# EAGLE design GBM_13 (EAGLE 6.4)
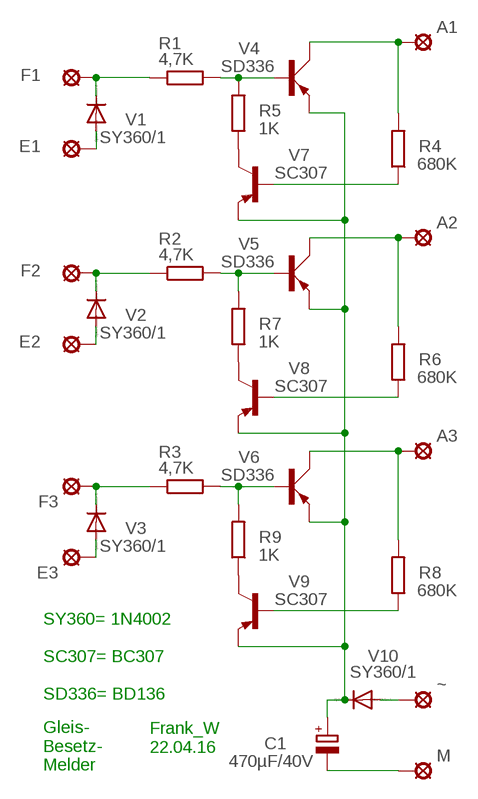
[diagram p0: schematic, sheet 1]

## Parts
A1  LSP10  [LSP10]
A2  LSP10  [LSP10]
A3  LSP10  [LSP10]
C1  470µF/40V  CPOL-EUE22-9AXIAL  [E22-9]
E1  LSP10  [LSP10]
E2  LSP10  [LSP10]
E3  LSP10  [LSP10]
F1  LSP10  [LSP10]
F2  LSP10  [LSP10]
F3  LSP10  [LSP10]
M  LSP10  [LSP10]
R1  4,7K  R-EU_0207/12  [0207/12]
R2  4,7K  R-EU_0207/12  [0207/12]
R3  4,7K  R-EU_0207/12  [0207/12]
R4  680K  R-EU_0207/12  [0207/12]
R5  1K  R-EU_0207/12  [0207/12]
R6  680K  R-EU_0207/12  [0207/12]
R7  1K  R-EU_0207/12  [0207/12]
R8  680K  R-EU_0207/12  [0207/12]
R9  1K  R-EU_0207/12  [0207/12]
V1  SY360/1  1N4004  [DO41-10]
V2  SY360/1  1N4004  [DO41-10]
V3  SY360/1  1N4004  [DO41-10]
V4  SD336  BD140  [TO126AV]
V5  SD336  BD140  [TO126AV]
V6  SD336  BD140  [TO126AV]
V7  SC307  BC307  [TO92]
V8  SC307  BC307  [TO92]
V9  SC307  BC307  [TO92]
V10  SY360/1  1N4004  [DO41-10]
~  LSP10  [LSP10]

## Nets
N$1: E1.MP V1.A
N$2: F1.MP R1.1 V1.C
N$3: R1.2 R5.2 V4.B
N$4: A1.MP R4.2 V4.C
N$5: R4.1 V7.2(B)
N$6: R5.1 V7.3(C)
N$7: F2.MP R2.1 V2.C
N$8: E2.MP V2.A
N$9: R2.2 R7.2 V5.B
N$10: R7.1 V8.3(C)
N$11: A2.MP R6.2 V5.C
N$12: R6.1 V8.2(B)
N$13: R9.1 V9.3(C)
N$14: F3.MP R3.1 V3.C
N$15: R3.2 R9.2 V6.B
N$16: A3.MP R8.2 V6.C
N$17: R8.1 V9.2(B)
N$18: E3.MP V3.A
N$19: V10.A ~.MP
N$20: C1.- M.MP
N$21: C1.+ V4.E V5.E V6.E V7.1(E) V8.1(E) V9.1(E) V10.C

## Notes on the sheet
- SY360= 1N4002
  
  SC307= BC307
  
  SD336= BD136
- Frank_W
  22.04.16
- Gleis-
  Besetz-
  Melder

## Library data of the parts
A1-A3 E1-E3 F1-F3 M ~ = solpad:LSP10: SOLDER PAD
C1 = rcl:CPOL-EU: POLARIZED CAPACITOR, European symbol
R1-R9 = rcl:R-EU_: RESISTOR, European symbol
V1-V3 V10 = diode:1N4004: DIODE
V4-V6 = transistor-power:BD140: PNP TRANSISTOR
V7-V9 = transistor-pnp:BC307: PNP Transistor

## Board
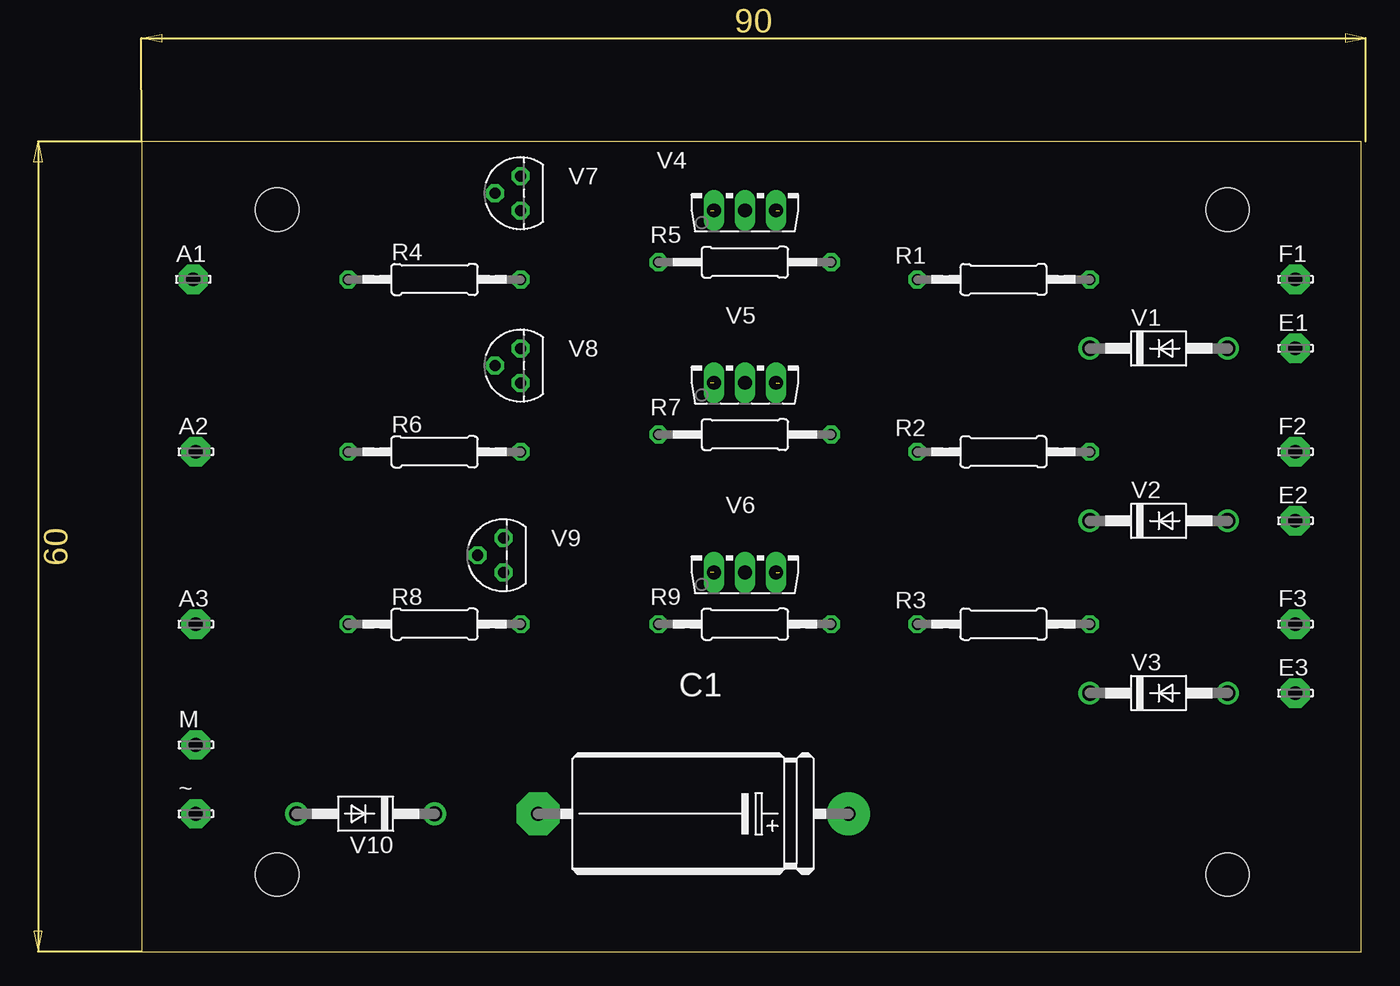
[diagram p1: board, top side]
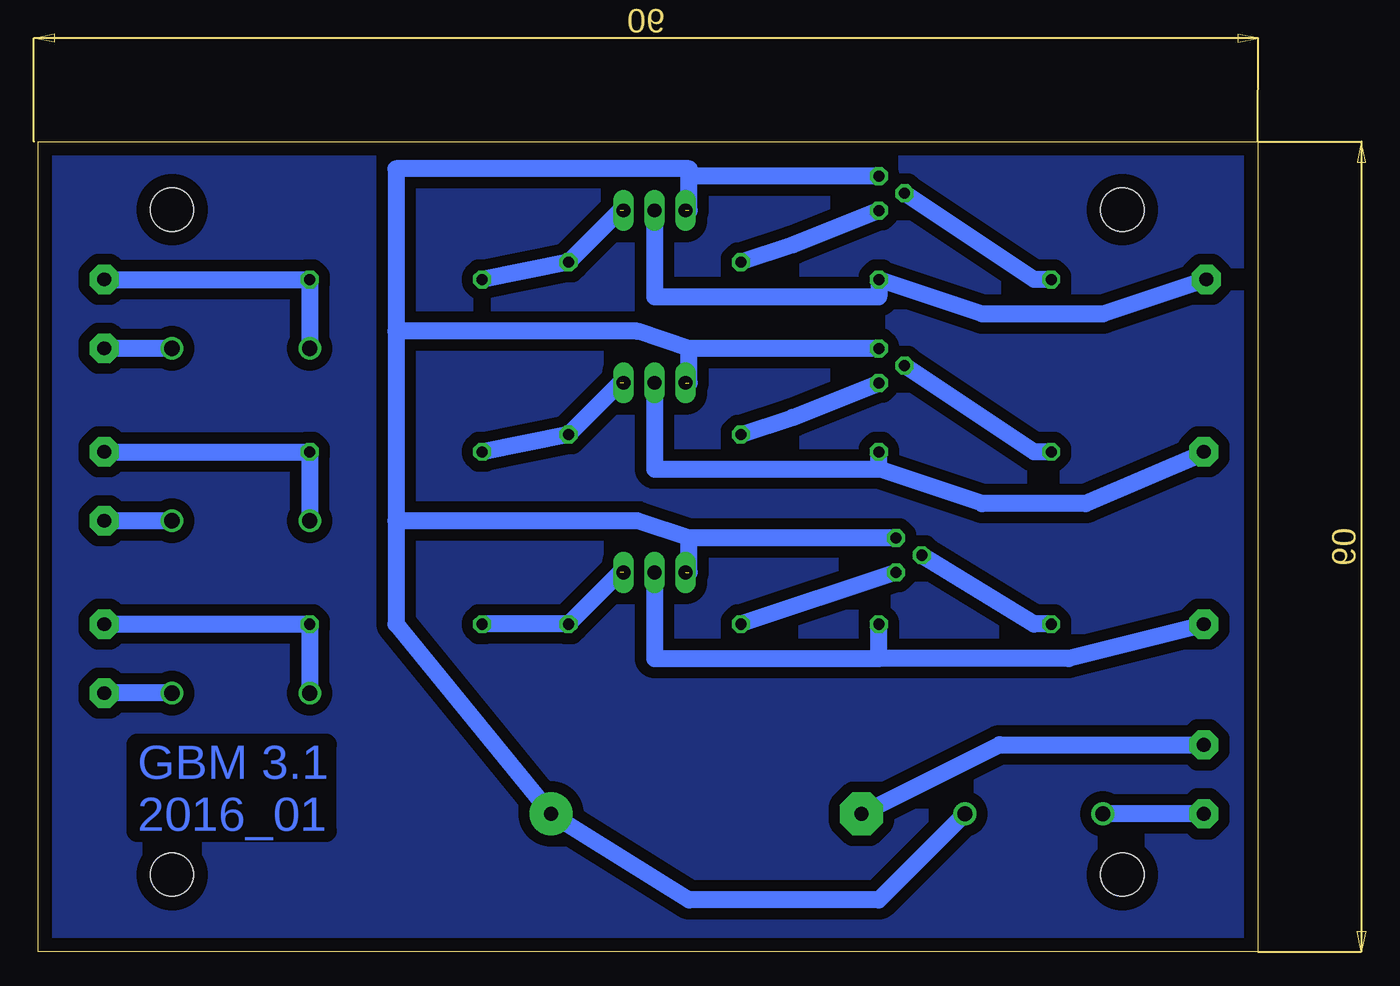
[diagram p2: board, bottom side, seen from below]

Size 98.09 x 67.61 mm. Coordinates in mm from the lower left corner, seen from the top.
Outline: 7.92,0 97.76,0 97.76,59.68 7.92,59.68 7.92,0
Copper layers (1*16): Top 0.035mm / dielectric 1.5mm / Bottom 0.035mm
Design rules "default *": minimum track width 20mil, minimum drill 24mil, track to track 8mil, track to pad 8mil, pad to pad 8mil, via to via 8mil, smd to smd 8mil, copper to edge 40mil, drill to drill 8mil, minimum pad ring 10mil, minimum via ring 8mil, stop-mask expansion 4mil, vias tented up to drill 0mil, thermal gap 20mil
Holes 3.2 mm at 87.92,54.68 87.92,5.68 17.92,5.68 17.92,54.68

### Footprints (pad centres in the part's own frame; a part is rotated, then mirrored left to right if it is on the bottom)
LSP10 = drill 1.016 pad 2.159 octagon: MP 0,0
E22-9 = drill 1.016 pad 3.15: + -11.43,0 | drill 1.016 pad 3.15 octagon: - 11.43,0
0207/12 = drill 0.813 octagon: 1 -6.35,0; 2 6.35,0
DO41-10 = drill 1.118: A 5.08,0; C -5.08,0
TO126AV = drill 1.016 long: B 2.286,-1.27; C 0,-1.27; E -2.286,-1.27
TO92 = drill 0.813 octagon: 1 1.27,0; 2 0,1.905; 3 -1.27,0

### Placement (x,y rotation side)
A1  11.73,49.53 0 top
A2  11.92,36.83 0 top
A3  11.92,24.13 0 top
C1  48.56,10.16 180 top
E1  92.92,44.45 0 top
E2  92.92,31.75 0 top
E3  92.92,19.05 0 top
F1  92.92,49.53 0 top
F2  92.92,36.83 0 top
F3  92.92,24.13 0 top
M  11.92,15.24 0 top
R1  71.42,49.53 180 top
R2  71.42,36.83 180 top
R3  71.42,24.13 180 top
R4  29.51,49.53 0 top
R5  52.37,50.8 0 top
R6  29.51,36.83 0 top
R7  52.37,38.1 0 top
R8  29.51,24.13 0 top
R9  52.37,24.13 0 top
V1  82.85,44.45 0 top
V2  82.85,31.75 0 top
V3  82.85,19.05 0 top
V4  52.37,55.88 0 top
V5  52.37,43.18 0 top
V6  52.37,29.21 0 top
V7  35.86,55.88 90 top
V8  35.86,43.18 90 top
V9  34.59,29.21 90 top
V10  24.43,10.16 180 top
~  11.92,10.16 0 top

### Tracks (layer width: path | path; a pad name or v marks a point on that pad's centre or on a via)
N$1
  Bottom 1.27: V1.A E1.MP
N$2
  Bottom 1.27: F1.MP R1.1 V1.C
N$3  (1 unrouted)
  Bottom 1.27: 54.91,54.61 R5.2 R1.2
N$4
  Bottom 1.27: A1.MP 19.35,46.99 28.24,46.99 R4.2 35.86,48.26 52.37,48.26 V4.C
N$5
  Bottom 1.27: R4.1 24.43,49.53 V7.2
N$6
  Bottom 1.27: V7.3 42.21,52.07 R5.1
N$7
  Bottom 1.27: F2.MP R2.1 V2.C
N$8
  Bottom 1.27: V2.A E2.MP
N$9  (1 unrouted)
  Bottom 1.27: 54.91,41.91 R7.2 R2.2
N$10
  Bottom 1.27: R7.1 42.21,39.37 V8.3
N$11
  Bottom 1.27: 35.86,35.56 52.37,35.56 V5.C | 35.86,35.56 R6.2 | A2.MP 11.73,36.83 20.62,33.02 28.24,33.02 35.86,35.56
N$12
  Bottom 1.27: R6.1 24.43,36.83 V8.2
N$13
  Bottom 1.27: V9.3 R9.1
N$14
  Bottom 1.27: F3.MP R3.1 V3.C
N$15  (1 unrouted)
  Bottom 1.27: 54.91,27.94 R9.2 R3.2
N$16
  Bottom 1.27: 35.86,21.59 52.37,21.59 V6.C | 35.86,21.59 R8.2 | A3.MP 11.73,24.13 21.89,21.59 35.86,21.59
N$17
  Bottom 1.27: R8.1 24.43,24.13 V9.2
N$18
  Bottom 1.27: V3.A E3.MP
N$19
  Bottom 1.27: ~.MP V10.A
N$20
  Bottom 1.27: C1.- 26.97,15.24 M.MP
N$21  (3 unrouted)
  Bottom 1.27: V10.C 35.86,3.81 49.83,3.81 C1.+ 71.42,24.13 71.42,31.75 | 49.83,54.61 49.83,57.15 | 71.42,45.72 71.42,57.68 49.83,57.68 49.83,57.15 | 71.42,45.72 71.42,31.75 | V7.1 49.83,57.15 | 49.83,41.91 49.83,44.45 | 49.83,44.45 53.64,45.72 71.42,45.72 | 49.83,27.94 49.83,30.48 | 49.83,30.48 53.64,31.75 71.42,31.75 | V8.1 49.83,44.45 | V9.1 49.83,30.48
N$22
  pour Bottom (isolate 0.813): 9.19,59.69 96.82,59.69 96.82,1.27 9.19,1.27

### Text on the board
Bottom: GBM 3.1 / 2016_01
